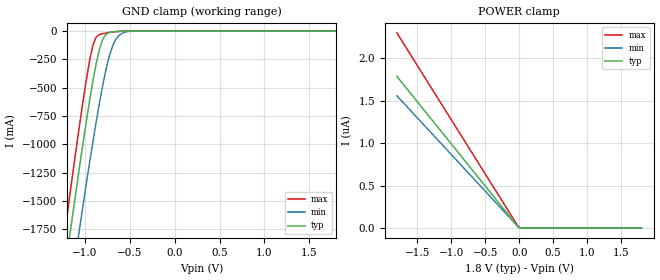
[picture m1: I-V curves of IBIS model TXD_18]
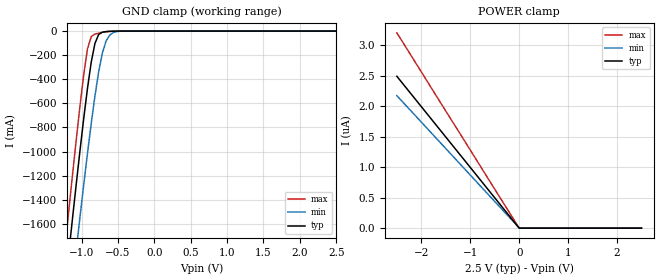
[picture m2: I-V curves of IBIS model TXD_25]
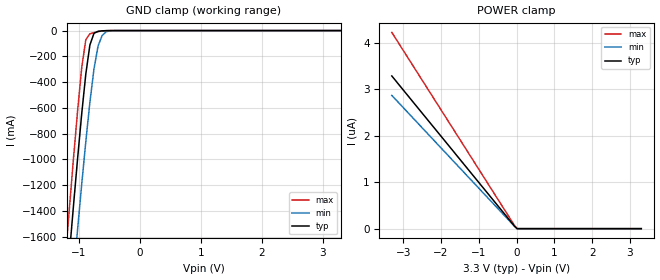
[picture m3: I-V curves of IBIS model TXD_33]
| IBIS file created by Layout Workbench Version 22.1.4.12161.401368   004
| Cadence Design Systems, Inc. 2011
[IBIS ver]   4.2
[File name]  iso6020.ibs
[File Rev]   1.5
[Date]   07 23, 2025
[Source]   Model built from TISPICED simulations at:
   Texas Instruments Incorporated.
   Analog-eLab, HPA 12500 TI Blvd
   Dallas, TX -75243
   For Support e-mail: elab_ibis@list.ti.com
[Notes]   This product is designed as an aid for customers of Texas Instruments.
   No warranties, either expressed or implied, with respect to this third party software (if any)
   or with respect to its fitness for any particular purpose is claimed by Texas Instruments or
   the author. The software (if any) is provided solely on an "as is" basis. The entire risk as to
   its quality and performance is with the customer
[Disclaimer]  This product is designed as an aid for customers of Texas Instruments. No warranties, either expressed or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
[Copyright] (C)Copyright 2025 Texas Instruments Incorporated. All rights reserved.
|   Component ISO60XX
[Component] ISO6020D
[Manufacturer] Texas Instruments Incorporated
[Package]   |16-pin SOIC DW package
|   typ   min   max
R_pkg   0.055   0.034   0.067
L_pkg   1.795nH   1.699nH   1.914nH
C_pkg   0.299pF   0.278pF   0.311pF
[Pin]   signal_name   model_name   R_pin   L_pin   C_pin
1   VCC1   POWER   0.067   1.914n   0.278p
2   INA   TXD1   0.062   1.816n   0.301p
3   INB   TXD1   0.053   1.699n   0.298p
4   GND1   GND   0.067   1.907n   0.278p
5   GND2   GND   0.034   1.704n   0.311p
6   OUTB   RXD2   0.061   1.808n   0.310p
7   OUTA   RXD2   0.062   1.817n   0.302p
8   VCC2   POWER   0.034   1.716n   0.311p
[Model Selector] TXD1
TXD_18   TXD Input model for 1.71V - 1.89V
TXD_25   TXD Input model for 2.25V - 2.75V
TXD_33   TXD Input model for 3.0V - 3.6V
TXD_5   TXD Input model for 4.5V - 5.5V
[Model Selector] RXD1
RXD_18   RXD Output model for 1.71V - 1.89V
RXD_25   RXD Output model for 2.25V - 2.75V
RXD_33   RXD Output model for 3.0V - 3.6V
RXD_5   RXD Output model for 4.5V - 5.5V
[Model Selector] TXD2
TXD_18   TXD Input model for 1.71V - 1.89V
TXD_25   TXD Input model for 2.25V - 2.75V
TXD_33   TXD Input model for 3.0V - 3.6V
TXD_5   TXD Input model for 4.5V - 5.5V
[Model Selector] RXD2
RXD_18   RXD Output model for 1.71V - 1.89V
RXD_25   RXD Output model for 2.25V - 2.75V
RXD_33   RXD Output model for 3.0V - 3.6V
RXD_5   RXD Output model for 4.5V - 5.5V
| Models and submodels in the file (8): TXD_18 (Input), TXD_25 (Input), TXD_33 (Input), TXD_5 (Input), RXD_18 (3-state), RXD_25 (3-state), RXD_33 (3-state), RXD_5 (3-state)
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|   TXD_18 Model
[Model]   TXD_18
Model_type   Input
|Signals   TXD
Vinl =  0.540V
Vinh =  1.260V
|   typ   min   max
C_comp   1.3pF   1.1pF   1.5pF
|   typ   min   max
[Temperature Range]   27   -55   150
[Voltage range]   1.8V   1.71V   1.89V
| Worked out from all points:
|   GND clamp passes 1 mA (typ) near -0.58 V on its own axis
[GND_clamp]
|Voltage   I(typ)   I(min)   I(max)
-1.8V     -5.506A    -5.93A     -5.269A
-1.245V   -2.234A    -2.756A    -1.895A
-1.208V   -2.022A    -2.55A     -1.676A
-1.171V   -1.811A    -2.345A    -1.459A
-1.06V    -1.194A    -1.742A    -825mA
-986mV    -801.2mA   -1.352A    -434mA
-912mV    -441.2mA   -978.2mA   -124.7mA
-838mV    -157.5mA   -630.6mA   -29.51mA
-764mV    -27.09mA   -331.9mA   -16.92mA
-690mV    -5.983mA   -125.6mA   -8.447mA
-542mV    -399.5uA   -6.689mA   -494.2uA
1.8V      0A         0A         -115nA
[POWER_clamp]
|Voltage   I(typ)   I(min)   I(max)
-1.8V     1.789uA    1.56uA     2.301uA
-13mV     12.95nA    15nA       16.65nA
24mV      0A         0A         0A
1.8V      0A         0A         0A
|   TXD_25 Model
[Model]   TXD_25
Model_type   Input
|Signals   TXD
Vinl =  0.750V
Vinh =  1.750V
|   typ   min   max
C_comp   1.3pF   1.1pF   1.5pF
|   typ   min   max
[Temperature Range]   27   -55   150
[Voltage range]   2.5V   2.25V   2.75V
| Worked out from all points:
|   GND clamp passes 1 mA (typ) near -0.58 V on its own axis
[GND_clamp]
|Voltage   I(typ)   I(min)   I(max)
-2.5V     -9.287A    -9.122A    -9.461A
-1.225V   -2.119A    -2.645A    -1.776A
-1.174V   -1.828A    -2.362A    -1.476A
-1.123V   -1.541A    -2.083A    -1.181A
-1.072V   -1.259A    -1.806A    -891.7mA
-1.021V   -984.1mA   -1.535A    -613.8mA
-919mV    -473.2mA   -1.013A    -146.1mA
-817mV    -102.7mA   -539.5mA   -24.7mA
-715mV    -9.204mA   -182mA     -10.99mA
-664mV    -3.989mA   -82.28mA   -6.169mA
-562mV    -642.2uA   -10.9mA    -884.6uA
2.5V      0A         0A         -319.8nA
[POWER_clamp]
|Voltage   I(typ)   I(min)   I(max)
-2.5V     2.488uA    2.171uA    3.199uA
1mV       0A         2.987nA    0A
52mV      0A         0A         0A
2.5V      0A         0A         0A
|   TXD_33 Model
[Model]   TXD_33
Model_type   Input
|Signals   TXD
Vinl =  0.990V
Vinh =  2.310V
|   typ   min   max
C_comp   1.3pF   1.1pF   1.5pF
|   typ   min   max
[Temperature Range]   27   -55   150
[Voltage range]   3.3V   3.0V   3.6V
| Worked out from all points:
|   GND clamp passes 1 mA (typ) near -0.57 V on its own axis
[GND_clamp]
|Voltage   I(typ)   I(min)   I(max)
-3.3V     -12.37A    -12.1A     -12.66A
-1.223V   -2.107A    -2.633A    -1.764A
-1.156V   -1.727A    -2.263A    -1.371A
-1.089V   -1.353A    -1.898A    -987mA
-1.022V   -989.5mA   -1.54A     -619.1mA
-955mV    -645mA     -1.193A    -287.8mA
-888mV    -337.4mA   -861.8mA   -70.28mA
-821mV    -112mA     -556.5mA   -25.45mA
-754mV    -21.16mA   -297.6mA   -15.62mA
-687mV    -5.702mA   -119.8mA   -8.165mA
-553mV    -522.6uA   -8.764mA   -688.5uA
3.3V      0A         0A         -383.9nA
[POWER_clamp]
|Voltage   I(typ)   I(min)   I(max)
-3.3V     3.286uA    2.868uA    4.224uA
-50mV     49.84nA    47.39nA    64.06nA
17mV      0A         0A         0A
3.3V      0A         0A         0A
